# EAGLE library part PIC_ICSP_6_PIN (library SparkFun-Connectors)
ISCP Programming connector for PICs This 6 pin header contains all the lines necessary for programming most PIC microcontrollers. Here is the connector we sell at SparkFun: Polarized Connectors - Header (6-Pin) (PRT-08094) It is used on this SparkFun product: SparkFun UDB5 - PIC UAV Development Board (DEV-11703) Also, if you need a nice PIC programmer, please check these out: MPLAB PICkit 3 (PGM-09973)
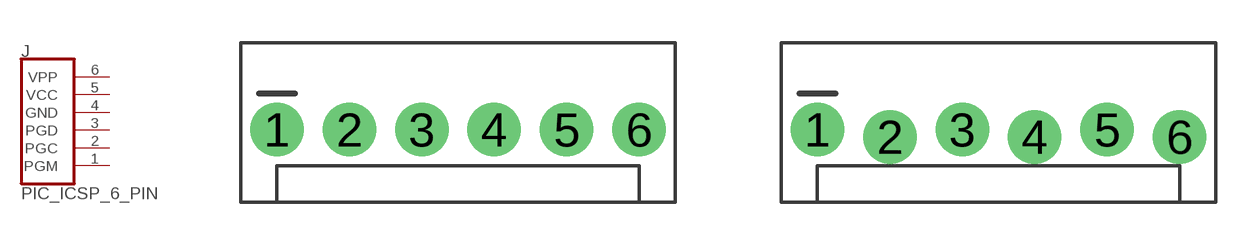
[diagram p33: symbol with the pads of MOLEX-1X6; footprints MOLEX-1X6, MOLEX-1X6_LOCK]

Designator prefix J

## PIC_ICSP_6_PIN (PROD_ID: CONN-08046; SF_ID: PRT-08094)  [MOLEX-1X6]
1  PGM
2  PGC
3  PGD
4  GND  pwr
5  VCC  pwr
6  VPP

## PIC_ICSP_6_PINPOLAR_LOCK  [MOLEX-1X6_LOCK]
Pads as for MOLEX-1X6

## Footprint MOLEX-1X6 (pad centres in mm)
Molex 6-Pin Plated Through-Hole Specifications: Pin count:6 Pin pitch:0.1" Datasheet referenced for footprint Example device(s): CONN_06
drill 1.016 pad 1.88: 1 0,0; 2 2.54,0; 3 5.08,0; 4 7.62,0; 5 10.16,0; 6 12.7,0

## Footprint MOLEX-1X6_LOCK (pad centres in mm)
Molex 6-Pin Plated Through-Hole Locking Footprint Holes are offset 0.005" from center to hold pins in place during soldering. Specifications: Pin count:6 Pin pitch:0.1" Datasheet referenced for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
drill 1.016 pad 1.88: 1 0,0; 2 2.54,-0.254; 3 5.08,0; 4 7.62,-0.254; 5 10.16,0; 6 12.7,-0.254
